FUNCTION_BLOCK Example05_pmccontrol //2x2 flyways w/ 1 xbots sample trajectory set as trajectory 1 (time interval = 10 ms) - trajectory, pause, resume, stop, deactivate, reboot, activate, levitate, arc center
VAR_INPUT
	Execute : BOOL;
END_VAR
VAR_OUTPUT
	Done : BOOL;
END_VAR
VAR_IN_OUT
	PM_Controller : PMControllerType;	// the planar motor controller to use
END_VAR
VAR
	PMC_XYMotion1 : PMC_XYMotion;
	xbotID_array12 : ARRAY[0..11] OF USINT;
	trajID_array12 : ARRAY[0..11] OF USINT;
	PMC_ActivateTrajectory1 : PMC_ActivateTrajectory;
	Delay1 : Delay;
	PMC_PauseXbots1 : PMC_PauseXbots;
	Delay2 : Delay;
	PMC_ResumeXbots1 : PMC_ResumeXbots;
	Delay3 : Delay;
	PMC_StopXbots1 : PMC_StopXbots;
	PMC_ArcMotionCenter1 : PMC_ArcMotionCenter;
	PMC_DeactivateXbots1 : PMC_DeactivateXbots;
	Delay4 : Delay;
	PMC_Reboot1 : PMC_Reboot;
	Delay5 : Delay;
	PMC_ActivateXbots1 : PMC_ActivateXbots;
	Delay6 : Delay;
	PMC_LevitationCtrl1 : PMC_LevitationCtrl;
	Delay7 : Delay;
	PMC_LevitationCtrl2 : PMC_LevitationCtrl;
END_VAR

//2x2 flyways w/ 1 xbots sample trajectory set as trajectory 1 (time interval = 10 ms) - trajectory, pause, resume, stop, deactivate, reboot, activate, levitate, arc center

//move xbot 1 to 240,240
PMC_XYMotion1(Execute := Execute,cmdLB := 1,XbotID := 1,Mode := 0,Type_ := 0,PosX := 0.24,PosY := 0.24,EndVel := 0,MaxVel := 1,MaxAcc := 10,PM_Controller := PM_Controller);

//xbot 1 does trajectory 1
xbotID_array12[0] := 1; trajID_array12[0] := 1;
PMC_ActivateTrajectory1(Execute := PMC_XYMotion1.Done,cmdLB := 2,nXbots := 1,XbotID := xbotID_array12,TrajID := trajID_array12,PM_Controller := PM_Controller);

Delay1(Execute := PMC_ActivateTrajectory1.Ack,Cycles := 5000);

//pause xbot 1
PMC_PauseXbots1(Execute := Delay1.Done,XbotID := 1,PM_Controller := PM_Controller);

Delay2(Execute := PMC_PauseXbots1.Done,Cycles := 5000);

//resume xbot 1
PMC_ResumeXbots1(Execute := Delay2.Done,XbotID := 1,PM_Controller := PM_Controller);

Delay3(Execute := PMC_ResumeXbots1.Done,Cycles := 4500);

//stop xbot 1
PMC_StopXbots1(Execute := Delay3.Done,XbotID := 1,PM_Controller := PM_Controller);

//360 around 240,240
PMC_ArcMotionCenter1(Execute := PMC_StopXbots1.Done,cmdLB := 6,XbotID := 1,Mode := 0,Dir := 0,EndVel := 0,MaxVel := 1,MaxAcc := 10,CenterX := 0.24,CenterY := 0.24,Angle := 6.283,PM_Controller := PM_Controller);

//deactivate PMC
PMC_DeactivateXbots1(Execute := PMC_ArcMotionCenter1.Done,PM_Controller := PM_Controller);

Delay4(Execute := PMC_DeactivateXbots1.Done,Cycles := 2000);

//reboot PMC
PMC_Reboot1(Execute := Delay4.Done,PM_Controller := PM_Controller);

Delay5(Execute := PMC_Reboot1.Done,Cycles := 2000);

//activate PMC
PMC_ActivateXbots1(Execute := Delay5.Done,PM_Controller := PM_Controller);

Delay6(Execute := PMC_ActivateXbots1.Done,Cycles := 2000);

//Land xbot 1
PMC_LevitationCtrl1(Execute := Delay6.Done,XbotID := 1,Level := 0,Speed := 0,LandedZForce := 0,PM_Controller := PM_Controller);

Delay7(Execute := PMC_LevitationCtrl1.Done,Cycles := 2000);

//Levitate xbot 1
PMC_LevitationCtrl2(Execute := Delay7.Done,XbotID := 1,Level := 1,Speed := 0,LandedZForce := 0,PM_Controller := PM_Controller);

Done := PMC_LevitationCtrl2.Done;

END_FUNCTION_BLOCK
